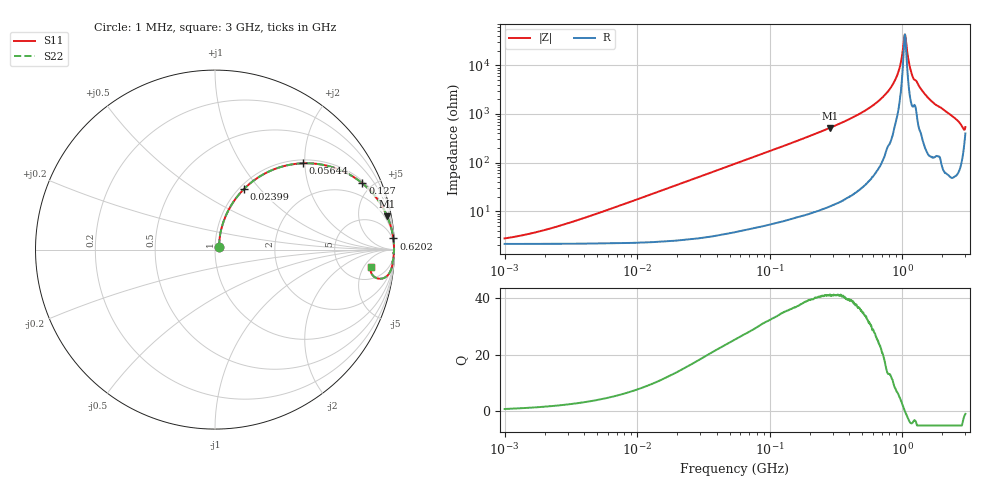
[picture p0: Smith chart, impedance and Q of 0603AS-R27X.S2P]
!s-Parameter Generated by FASTRON Sdn. Bhd.
!FASTRON P/N : 0603AS-R27X
!Keysight Technologies: E4991B_MY54100416_A.01.15
!Date created: Tue Oct 17 15:19:06 2023
!Version  : Rev01 Tue Oct 17 15:19:06 2023
!Data & Calibration Information:
!Freq	S11	S21	S12	S22
!PortZ  Port1:50+j0  Port2:50+j0
!When reading reference impedance value at option line is always used.
! Remarks : This data is being provided solely for informational purposes.
# Hz S dB R 50
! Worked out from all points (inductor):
!   1601 points, 1 MHz to 3 GHz, reference 50 ohm
!   read as one part in series: L = 278 nH near 3.71 MHz
!   highest Q = 41.1 at 284.1 MHz (marker M1), where L = 289 nH
!   self-resonance near 1.049 GHz
!   S11 on the Smith chart (normalised r, x): 1 MHz: 1.04, +0.04; 23.99 MHz: 1.05, +0.83; 56.44 MHz: 1.08, +1.95; 127 MHz: 1.13, +4.39; 620.2 MHz: 2, +32; 3 GHz: 9, -7
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1000000  -31.33 38.5  -0.19 -1.0  -0.19 -1.0  -31.33 38.5
3804036  -23.30 68.3  -0.20 -3.7  -0.20 -3.7  -23.30 68.3
1.447069e7  -12.40 70.8  -0.46 -13.8  -0.46 -13.8  -12.40 70.8
2.398736e7  -8.48 64.3  -0.89 -22.1  -0.89 -22.1  -8.48 64.3
5.477226e7  -3.42 45.4  -2.94 -42.3  -2.94 -42.3  -3.42 45.4
5.644167e7  -3.29 44.6  -3.07 -43.2  -3.07 -43.2  -3.29 44.6
1.269575e8  -0.91 24.2  -7.74 -64.1  -7.74 -64.1  -0.91 24.2
2.083556e8  -0.37 15.1  -11.66 -73.4  -11.66 -73.4  -0.37 15.1
2.841474e8  -0.20 10.9  -14.46 -77.7  -14.46 -77.7  -0.20 10.9
6.202446e8  -0.04 3.6  -24.08 -84.4  -24.08 -84.4  -0.04 3.6
7.925923e8  -0.03 1.9  -29.69 -83.8  -29.69 -83.8  -0.03 1.9
9.255909e8  -0.02 0.8  -36.51 -80.4  -36.51 -80.4  -0.02 0.8
9.682285e8  -0.02 0.5  -40.18 -76.7  -40.18 -76.7  -0.02 0.5
1.023018e9  -0.02 0.2  -48.47 -53.3  -48.47 -53.3  -0.02 0.2
1.054198e9  -0.02 -0.0  -52.42 12.1  -52.42 12.1  -0.02 -0.0
1.075512e9  -0.02 -0.2  -48.61 50.8  -48.61 50.8  -0.02 -0.2
1.136371e9  -0.02 -0.6  -40.00 74.0  -40.00 74.0  -0.02 -0.6
1.188719e9  -0.03 -0.9  -35.98 75.6  -35.98 75.6  -0.03 -0.9
1.402151e9  -0.04 -1.8  -29.96 81.8  -29.96 81.8  -0.04 -1.8
1.712864e9  -0.05 -3.3  -24.71 82.4  -24.71 82.4  -0.05 -3.3
2.568929e9  -0.15 -7.3  -17.86 78.5  -17.86 78.5  -0.15 -7.3
3e9  -1.17 -6.3  -15.79 35.9  -15.79 35.9  -1.17 -6.3
